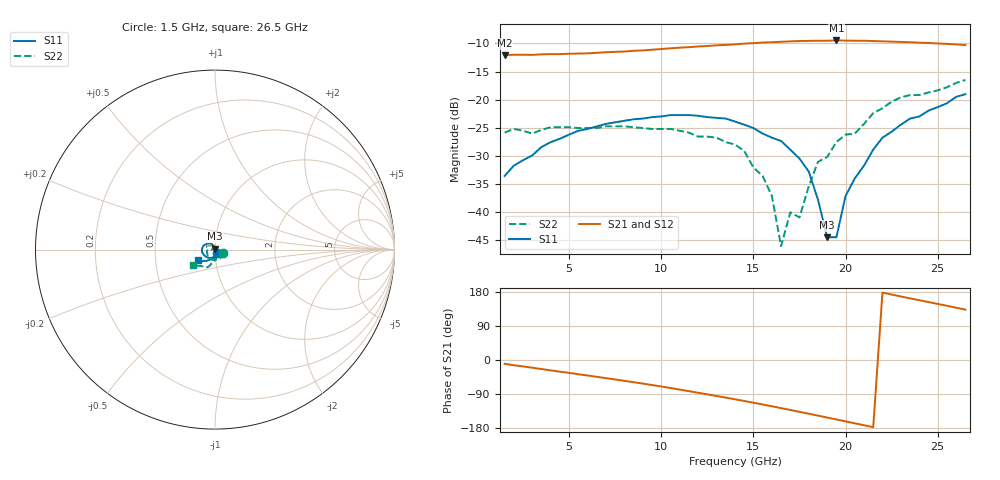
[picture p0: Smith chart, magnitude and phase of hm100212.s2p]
! HMMC-1002
! S-PARAMETERS at 12 dB attenuation setting. LAST UPDATED  07-06-99
# GHZ  S  MA  R  50
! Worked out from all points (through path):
!   51 points, 1.5 GHz to 26.5 GHz, reference 50 ohm
!   highest |S21| = -9.47 dB at 19.5 GHz (marker M1); lowest = -12.1 dB at 1.5 GHz (marker M2)
!   group delay of S21, straight-line fit = 24.4 ps
!   lowest |S11| = -44.4 dB at 19 GHz (marker M3), VSWR 1.01, Z = 50.2 + j0.579 ohm
!   |S11| at or under -10 dB: start of sweep to end of sweep
!   |S22| runs from -46.0 to -16.5 dB; largest |S21 - S12| = 0.0054
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1.5  0.021 -53.9  0.249 -10.1  0.249 -10.5  0.051 -22.8
3.5  0.038 -89.4  0.253 -23.8  0.253 -24.1  0.054 -51.2
6  0.055 -123.2  0.258 -40.9  0.258 -41.1  0.056 -87.5
10  0.071 -162.2  0.282 -69.9  0.282 -70.1  0.055 -132.7
14  0.064 155.8  0.31 -103.7  0.31 -103.6  0.04 -176.7
14.5  0.06 151.2  0.315 -108.1  0.314 -108.1  0.035 177.2
15  0.056 144.3  0.318 -112.7  0.318 -112.7  0.025 178.3
15.5  0.05 138.8  0.322 -117.4  0.322 -117.4  0.021 -178.2
16  0.046 135.2  0.324 -122.1  0.324 -122.1  0.014 166.1
16.5  0.043 126.6  0.327 -127.0  0.327 -126.9  0.005 -161.7
17  0.036 119.8  0.33 -131.8  0.329 -131.8  0.01 -132.9
17.5  0.03 117.1  0.332 -136.8  0.331 -136.7  0.009 -125.9
18  0.023 107.4  0.333 -141.7  0.333 -141.6  0.017 -82.1
18.5  0.013 93.7  0.334 -146.8  0.334 -146.7  0.028 -86.3
19  0.006 74.0  0.334 -151.8  0.335 -151.6  0.031 -82.5
19.5  0.006 -15.1  0.336 -156.9  0.335 -156.6  0.042 -74.4
20  0.014 -61.0  0.335 -161.9  0.334 -161.6  0.049 -83.5
20.5  0.02 -81.5  0.334 -167.1  0.334 -166.8  0.05 -87.5
21.5  0.036 -92.9  0.332 -177.2  0.332 -176.9  0.076 -100.1
22.5  0.052 -108.7  0.328 172.7  0.329 173.2  0.096 -108.5
23.5  0.068 -119.8  0.324 162.6  0.323 163.1  0.11 -116.2
26.5  0.112 -147.8  0.306 133.0  0.307 134.0  0.15 -143.9
